VAR_GLOBAL CONSTANT
		N_AXES			: USINT := 2;
	END_VAR
	VAR_GLOBAL
		gCommunicationReady	: BOOL := FALSE; (* Global indicator for Tria-Link and axes readiness *)
		gReset				: BOOL := FALSE; (* Global handle to reset axes errors *)
		gEnable				: BOOL := FALSE; (* Global handle to enable/disable axes *)
		
		gHli				: MCV_HliInterface;
		gTrialink			: Triamec.TL_Trialink2; (* The Trialink adapter *)
		gAxes				: ARRAY [1..N_AXES] OF Triamec.TL_Axis2; (* The Triamec Axis objects *)
		{attribute 'contextName' := 'TASK_FAST'}
		gCncAxes   			: ARRAY [1..N_AXES] OF TL_CNC_Axis; (* Link to the CNC pathplanner *)
		
		motorTemperature1	: Triamec.TL_MC_RegisterRead;
		publish1			: Triamec.TL_publishSlave2Master;
	END_VAR
